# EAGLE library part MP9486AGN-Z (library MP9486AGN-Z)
Switching Voltage Regulators 100V Input, 3.5A, Switching Current Limit Step-Down Converter Source: Datasheet
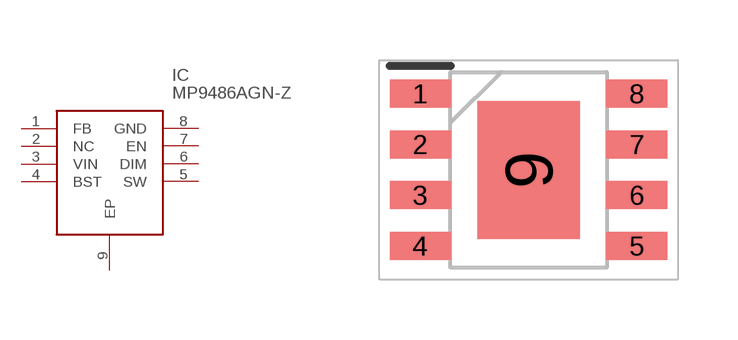
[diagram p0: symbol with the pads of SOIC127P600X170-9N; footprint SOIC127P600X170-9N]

Designator prefix IC

## MP9486AGN-Z (Description: Switching Voltage Regulators 100V Input, 3.5A, Switching Current Limit Step-Down Converter; Height: 1.7mm; Manufacturer_Name: Monolithic Power Systems (MPS); Manufacturer_Part_Number: MP9486AGN-Z; Mouser_Part_Number: 946-MP9486AGN-Z; Mouser_Price-Stock: https://www.mouser.co.uk/ProductDetail/Monolithic-Power-Systems-MPS/MP9486AGN-Z?qs=YCa%2FAAYMW010ws20lFESXg%3D%3D)  [SOIC127P600X170-9N]
1  FB
2  NC  nc
3  VIN
4  BST
5  SW
6  DIM
7  EN
8  GND
9  EP

## Footprint SOIC127P600X170-9N (pad centres in mm)
SOIC8 +
smd 1.525 x 0.7: 1 -2.712,1.905; 2 -2.712,0.635; 3 -2.712,-0.635; 4 -2.712,-1.905; 5 2.712,-1.905; 6 2.712,-0.635; 7 2.712,0.635; 8 2.712,1.905
smd 2.56 x 3.45: 9 0,0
